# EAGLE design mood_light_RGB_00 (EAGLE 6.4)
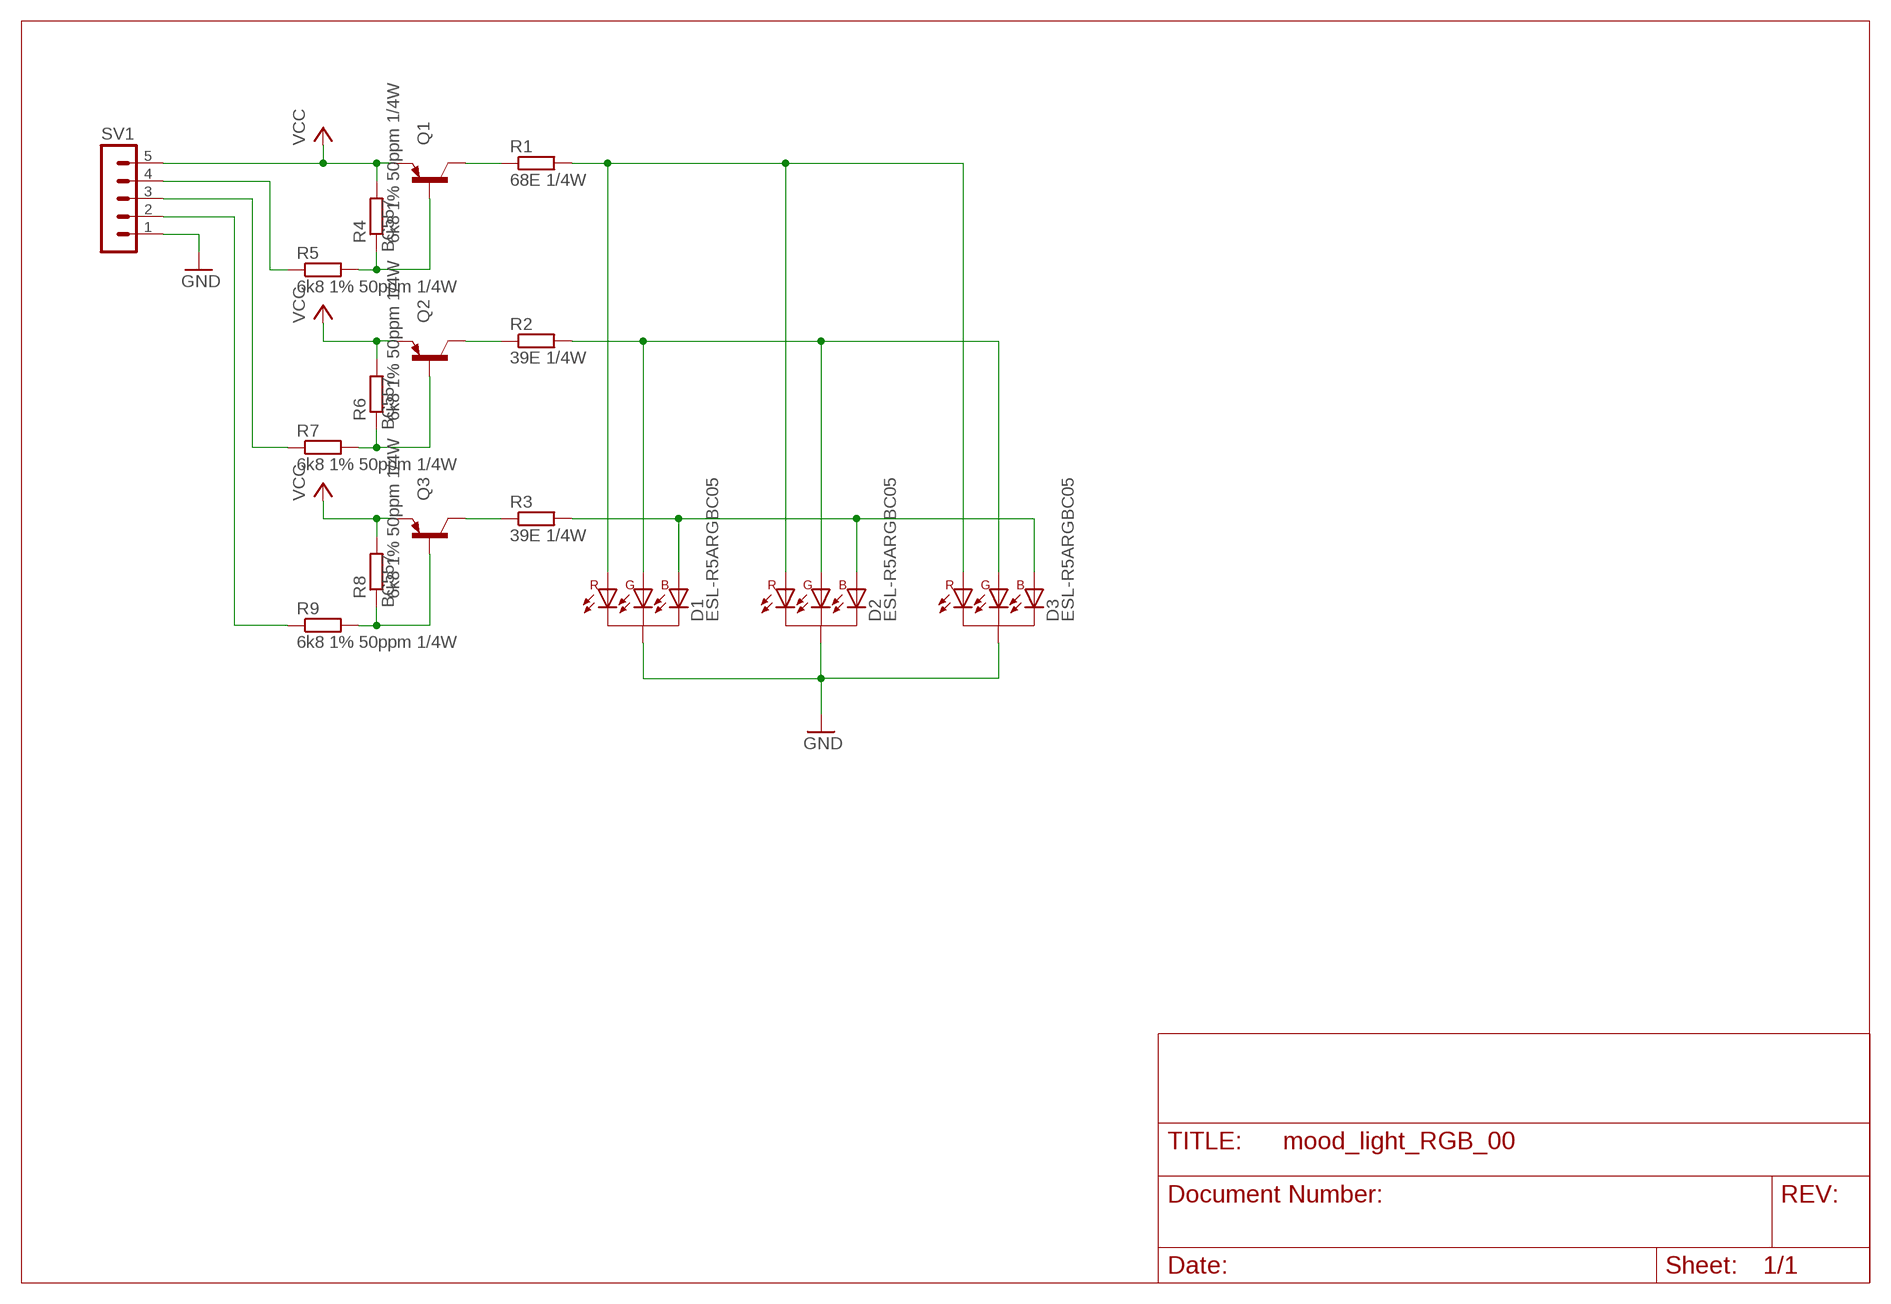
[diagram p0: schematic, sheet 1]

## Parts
D1  ESL-R5ARGBC05  [RGBLED-C-5MM]
D2  ESL-R5ARGBC05  [RGBLED-C-5MM]
D3  ESL-R5ARGBC05  [RGBLED-C-5MM]
Q1  BC557  [TO92-EBC]
Q2  BC557  [TO92-EBC]
Q3  BC557  [TO92-EBC]
R1  68E 1/4W  R-EU_0207/10  [0207/10]
R2  39E 1/4W  R-EU_0207/10  [0207/10]
R3  39E 1/4W  R-EU_0207/10  [0207/10]
R4  6k8 1% 50ppm 1/4W  R-EU_0207/10  [0207/10]
R5  6k8 1% 50ppm 1/4W  R-EU_0207/10  [0207/10]
R6  6k8 1% 50ppm 1/4W  R-EU_0207/10  [0207/10]
R7  6k8 1% 50ppm 1/4W  R-EU_0207/10  [0207/10]
R8  6k8 1% 50ppm 1/4W  R-EU_0207/10  [0207/10]
R9  6k8 1% 50ppm 1/4W  R-EU_0207/10  [0207/10]
SV1  MA05-1  [MA05-1]

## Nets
GND: D1.C D2.C D3.C SV1.1
N$1: Q1.C R1.1
N$2: Q2.B R6.1 R7.2
N$3: D1.AR D2.AR D3.AR R1.2
N$4: D1.AG D2.AG D3.AG R2.2
N$5: D1.AB D2.AB D3.AB R3.2
N$6: Q3.B R8.1 R9.2
N$7: Q2.C R2.1
N$8: Q3.C R3.1
N$9: Q1.B R4.1 R5.2
N$10: R5.1 SV1.4
N$17: R7.1 SV1.3
N$22: R9.1 SV1.2
VCC: Q1.E Q2.E Q3.E R4.2 R6.2 R8.2 SV1.5

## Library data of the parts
D1-D3 = optos:ESL-R5ARGBC05: EVERSTAR RGB LED Lichtfarbe: RGB Stromaufnahme: 65 mA Durchmesser: 5 mm Form: rund Gehäusefarbe: wasserklar Abstrahlwinkel: 60° Wellenlänge bei 1,8...2,4 V: 620...630 nm (rot) Lichtstärke: 20...28 mcd Wellenlänge bei 3,0...3,6 V: 510...525 nm (grün) Lichtstärke: 120...150 mcd Wellenlänge bei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
Q1-Q3 = transistor-pnp:BC557*: PNP Transistror
R1-R9 = rcl:R-EU_: RESISTOR, European symbol; OC_REICHELT: 1/4W; PART_VALUE: 1/4W 5%
SV1 = con-lstb:MA05-1: PIN HEADER; OC_FARNELL: unknown; OC_NEWARK: unknown

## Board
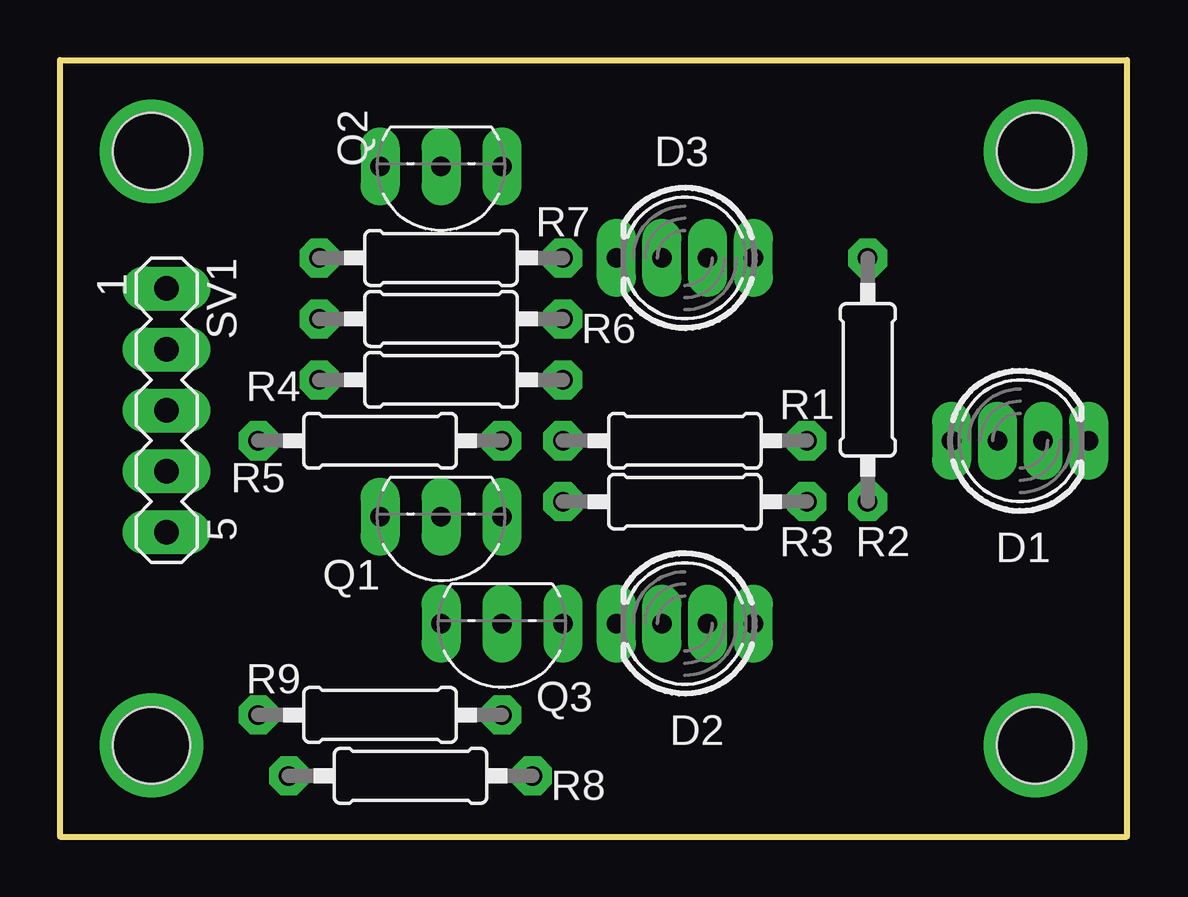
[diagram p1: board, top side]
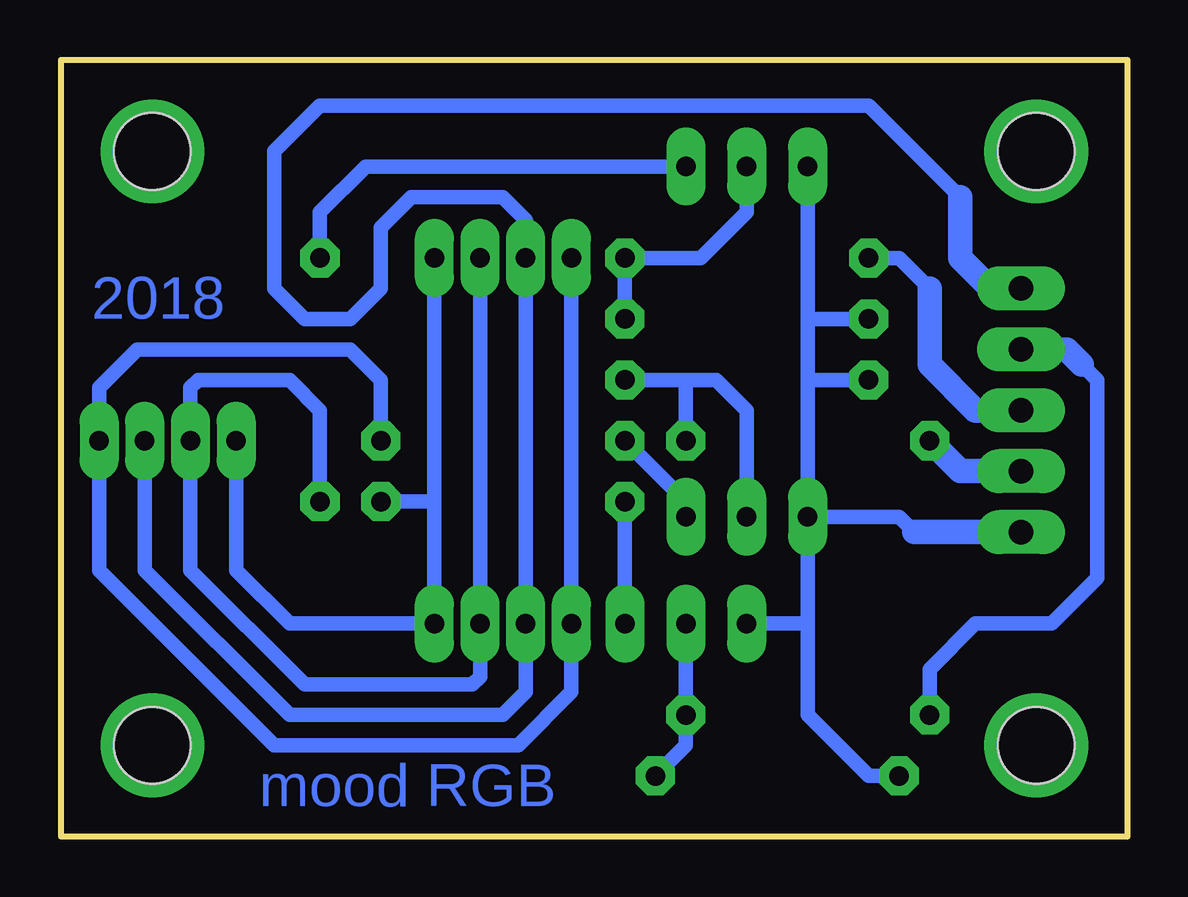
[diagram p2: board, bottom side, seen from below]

Size 44.45 x 32.38 mm. Coordinates in mm from the lower left corner, seen from the top.
Outline: 0,0 0,32.38 44.45,32.38 44.45,0 0,0
Copper layers (1*16): Top 0.035mm / dielectric 1.5mm / Bottom 0.035mm
Design rules "later_toner_transfer *": minimum track width 10mil, minimum drill 24mil, track to track 18mil, track to pad 18mil, pad to pad 18mil, via to via 18mil, smd to smd 18mil, copper to edge 40mil, drill to drill 16mil, minimum pad ring 16mil, minimum via ring 16mil, stop-mask expansion 4mil, vias tented up to drill 0mil, thermal gap 10mil
Holes 3.2 mm at 3.81,3.81 40.64,3.81 3.81,28.57 40.64,28.57

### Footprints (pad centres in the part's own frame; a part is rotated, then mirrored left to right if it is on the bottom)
RGBLED-C-5MM = drill 0.813 long: AB 2.857,0; AG 0.953,0; AR -2.857,0; C -0.953,0
TO92-EBC = drill 0.813 long: B 0,-1.27; C -2.54,-1.27; E 2.54,-1.27
0207/10 = drill 0.813 octagon: 1 -5.08,0; 2 5.08,0
MA05-1 = drill 1.016 long: 1 -5.08,0; 2 -2.54,0; 3 0,0; 4 2.54,0; 5 5.08,0

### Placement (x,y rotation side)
D1  40.01,16.51 180 top
D2  26.04,8.89 0 top
D3  26.04,24.13 0 top
Q1  15.88,12.06 180 top
Q2  15.88,26.67 180 top
Q3  18.41,7.62 180 top
R1  26.04,16.51 0 top
R2  33.66,19.05 270 top
R3  26.04,13.97 0 top
R4  15.88,19.05 180 top
R5  13.34,16.51 0 top
R6  15.88,21.59 180 top
R7  15.88,24.13 0 top
R8  14.61,2.54 180 top
R9  13.34,5.08 0 top
SV1  4.45,17.78 270 top

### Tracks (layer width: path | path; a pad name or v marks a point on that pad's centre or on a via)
GND
  Bottom 0.61: D1.C 40.96,11.11 34.92,5.08 26.04,5.08 25.08,6.03 D2.C D3.C 25.08,25.72 26.04,26.67 29.84,26.67 31.11,25.4 31.11,22.86 32.38,21.59 34.29,21.59 35.56,22.86 35.56,28.57 33.66,30.48 10.79,30.48 6.99,26.67
  Bottom 1.016: 6.99,26.67 6.99,24.13 5.71,22.86 SV1.1
N$1
  Bottom 0.61: R1.1 18.41,13.97 Q1.C
N$2
  Bottom 0.61: R6.1 R7.2 17.78,24.13 15.88,26.04 Q2.B
N$3
  Bottom 0.61: D3.AR D2.AR 23.18,6.03 25.4,3.81 35.56,3.81 42.86,11.11 D1.AR 42.86,18.73 41.27,20.32 32.38,20.32 31.11,19.05 R1.2
N$4
  Bottom 0.61: D3.AG D2.AG 26.99,6.67 27.3,6.35 34.29,6.35 39.05,11.11 D1.AG 39.05,18.73 38.73,19.05 34.92,19.05 33.66,17.78 R2.2
N$5
  Bottom 0.61: D1.AB 37.15,11.11 34.92,8.89 D2.AB 28.89,13.97 | 28.89,13.97 D3.AB | R3.2 28.89,13.97
N$6
  Bottom 0.61: Q3.B R9.2 18.41,3.81 R8.1
N$7
  Bottom 0.61: R2.1 33.66,26.04 31.75,27.94 Q2.C
N$8
  Bottom 0.61: Q3.C R3.1
N$9
  Bottom 0.61: Q1.B 15.88,17.78 17.14,19.05 18.41,19.05 | R5.2 18.41,19.05 | 18.41,19.05 R4.1
N$10
  Bottom 1.016: SV1.4 6.99,15.24 R5.1
N$11  (via drill 3.2 pad 3.81)
  other vias: 3.81,3.81
N$12  (via drill 3.2 pad 3.81)
  other vias: 40.64,3.81 40.64,28.57
N$13  (via drill 3.2 pad 3.81)
  other vias: 3.81,28.57
N$17
  Bottom 0.61: R7.1 9.53,24.13 8.26,22.86
  Bottom 1.016: 8.26,22.86 8.26,19.68 6.35,17.78 SV1.3
N$22
  Bottom 0.61: 1.91,19.68 1.27,19.05 1.27,10.79 3.17,8.89 6.35,8.89 8.26,6.99 R9.1
  Bottom 1.016: SV1.2 2.54,20.32 1.91,19.68
VCC
  Bottom 0.61: 13.34,21.59 R6.2 | 13.34,19.05 Q1.E | R8.2 10.79,2.54 13.34,5.08 13.34,8.89 | Q1.E 13.34,8.89 | Q3.E 13.34,8.89 | 8.89,12.7 9.53,13.34 Q1.E | R4.2 13.34,19.05 | 13.34,19.05 13.34,21.59 | 13.34,21.59 Q2.E
  Bottom 1.016: SV1.5 8.89,12.7

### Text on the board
Bottom: 2018 | mood RGB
